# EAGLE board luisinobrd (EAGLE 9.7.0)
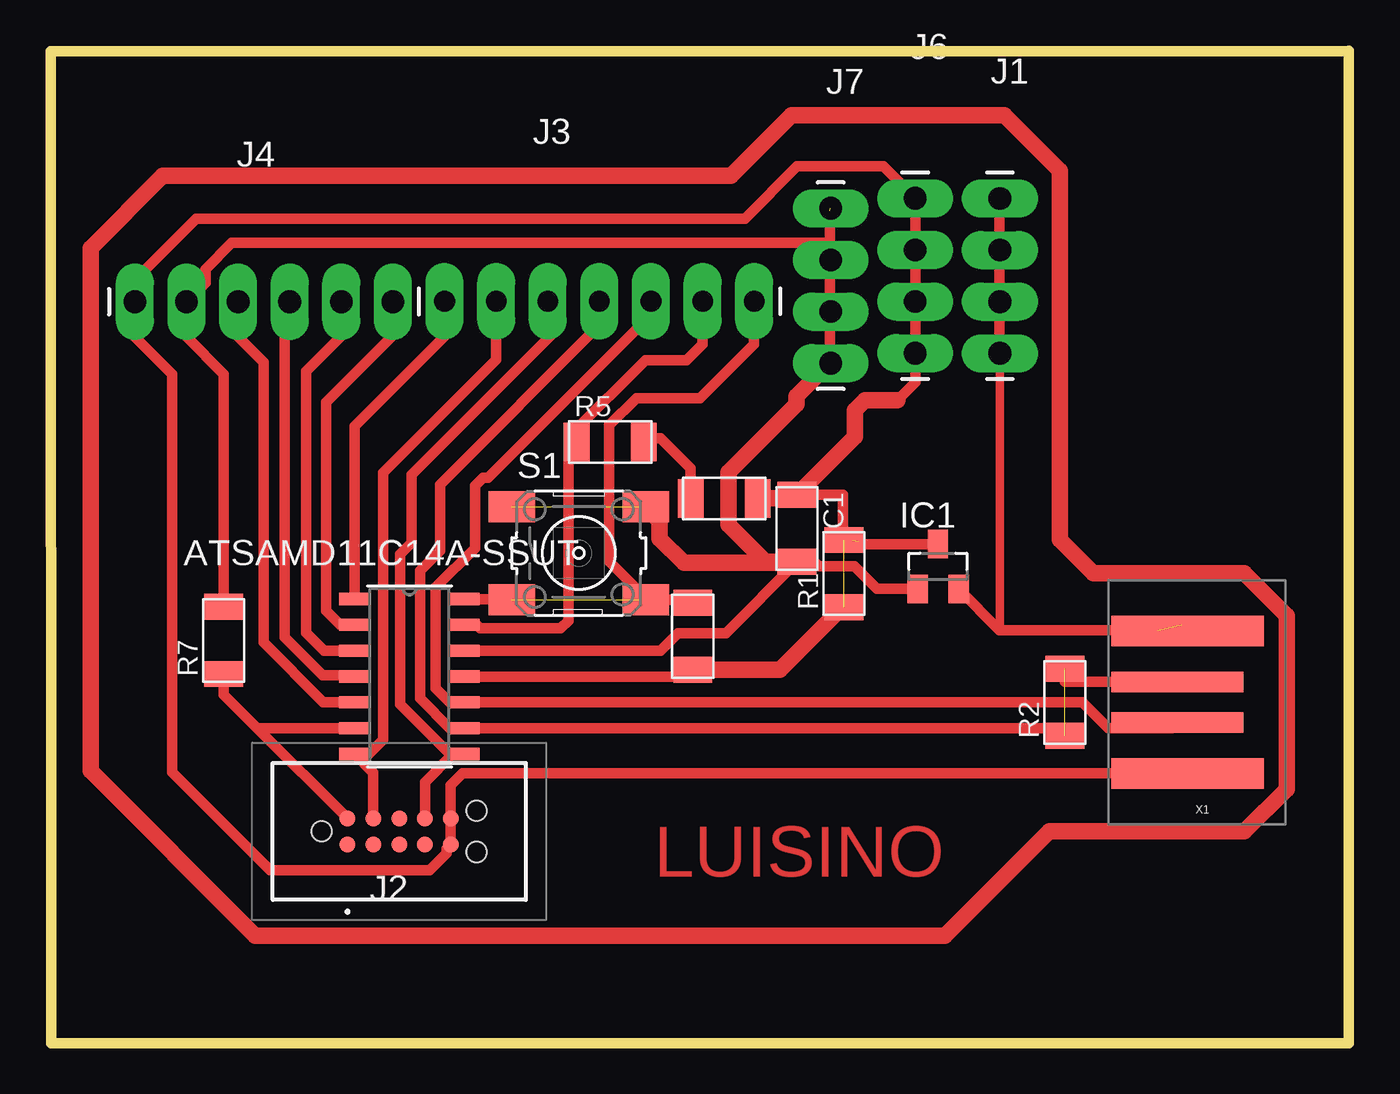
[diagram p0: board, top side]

Size 63.88 x 48.82 mm. Coordinates in mm from the lower left corner, seen from the top.
Outline: 63.88,48.82 63.88,0 0.02,0 0,48.79 63.88,48.79
Copper layers (1*16): Top / Bottom
Stack-up Default Layer Stack: Top User Defined 0.035mm / Dielectric-1 User Defined 1.5mm / Bottom User Defined 0.035mm
Design rules "default *": minimum track width 16mil, minimum drill 0.35mm, track to track 10mil, track to pad 16mil, pad to pad 16mil, via to via 16mil, smd to smd 6mil, copper to edge 16mil, drill to drill 16mil, minimum pad ring 10mil, minimum via ring 8mil, stop-mask expansion 4mil, vias tented up to drill 0mil, thermal gap 10mil

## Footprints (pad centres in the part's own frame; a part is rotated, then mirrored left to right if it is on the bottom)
C1206FAB = smd 1.27 x 1.905: 1 -1.651,0; 2 1.651,0
SOT23 = smd 1 x 1.4: 1 -1.001,-1.1; 2 1.014,-1.1; 3 0,1.1
1X04_LONGPADS = drill 1.118 pad 1.88 long: 1 0,0; 2 2.54,0; 3 5.08,0; 4 7.62,0
TC2050IDCNL = smd 0.787 x 0.787: 1 -2.54,-0.635; 2 -1.27,-0.635; 3 0,-0.635; 4 1.27,-0.635; 5 2.54,-0.635; 6 2.54,0.635; 7 1.27,0.635; 8 0,0.635; 9 -1.27,0.635; 10 -2.54,0.635 | hole 0.991: -3.81,0; 3.81,-1.015; 3.81,1.015
1X07_LONGPADS = drill 1.016 pad 1.88 long: 1 0,0; 2 2.54,0; 3 5.08,0; 4 7.62,0; 5 10.16,0; 6 12.7,0; 7 15.24,0
1X06_LONGPADS = drill 1.118 pad 1.88 long: 1 0,0; 2 2.54,0; 3 5.08,0; 4 7.62,0; 5 10.16,0; 6 12.7,0
R1206FAB = smd 1.27 x 1.905: 1 -1.651,0; 2 1.651,0
6MM_SWITCH = smd 2.286 x 1.524: 1 -3.302,2.286; 2 3.302,2.286; 3 -3.302,-2.286; 4 3.302,-2.286
SOIC14_SL_MCH = smd 1.5 x 0.6: 1 -2.7,3.81; 2 -2.7,2.54; 3 -2.7,1.27; 4 -2.7,0; 5 -2.7,-1.27; 6 -2.7,-2.54; 7 -2.7,-3.81; 8 2.7,-3.81; 9 2.7,-2.54; 10 2.7,-1.27; 11 2.7,0; 12 2.7,1.27; 13 2.7,2.54; 14 2.7,3.81
LED1206FAB = smd 1.27 x 1.905: 1 -1.651,0; 2 1.651,0
USB-A-PCB = smd 7.5 x 1.5: 5V -0.2,-3.5; GND -0.2,3.5 | smd 6.5 x 1: USB_M 0.3,-1; USB_P 0.3,1

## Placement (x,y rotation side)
C1  1uF  [C1206FAB]  36.73,25.32 270 top
IC1  [SOT23]  43.66,23.44 0 top
J1  [1X04_LONGPADS]  46.71,41.55 270 top
J2  TC2050-IDC-NL  [TC2050IDCNL]  17.14,10.41 0 top
J3  [1X07_LONGPADS]  19.38,36.5 0 top
J4  [1X06_LONGPADS]  4.14,36.47 0 top
J6  [1X04_LONGPADS]  42.55,41.56 270 top
J7  [1X04_LONGPADS]  38.38,41.07 270 top
R1  0  [R1206FAB]  39.04,23.1 90 top
R2  0  [R1206FAB]  49.91,16.76 90 top
R5  470  [R1206FAB]  27.53,29.57 0 top
R6  1k  [R1206FAB]  31.6,20.02 270 top
R7  10K  [R1206FAB]  8.51,19.81 90 top
S1  [6MM_SWITCH]  25.98,24.1 0 top
U1  ATSAMD11C14A-SSUT  [SOIC14_SL_MCH]  17.65,18.03 0 top
U$4  LEDFAB1206  [LED1206FAB]  33.15,26.8 0 top
X1  CONN_USBPCB  [USB-A-PCB]  55.75,16.76 180 top

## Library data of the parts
C1 IC1 R1 R2 R5-R7 S1 U$4 X1 = fab
J1 J6 J7 = SparkFun-Connectors; PROD_ID: CONN-09696
J2 = TC2050-IDC-NL; DESCRIPTION: 10-Pin No-Legs Plug-of-Nails Cable with Ribbon connector. CBL PLUG-OF-NAILS 10-PIN; HEIGHT: 29.66mm; MANUFACTURER_NAME: Tag-Connect; MANUFACTURER_PART_NUMBER: TC2050-IDC-NL
J3 J4 = SparkFun-Connectors
U1 = samd11c; BUILT_BY: EMA_Molly; COPYRIGHT: Copyright (C) 2018 Accelerated Designs. All rights reserved; MANUFACTURER_PART_NUMBER: ATSAMD11C14A-SSUT; SOURCELIBRARY: Microchip_2019-08-23_25; VENDOR: Microchip

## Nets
2: J3.6 R5.1 U1.13
4: J3.7 R6.1 S1.3 S1.4 U1.14
5: J3.1 U1.1
5V: IC1.2 J1.1 J1.2 J1.3 J1.4 X1.5V
8: J4.6 U1.2
9: J4.5 U1.3
24-: J3.4 R2.1 R2.2 U1.9 X1.USB_M
25+: J3.5 U1.10 X1.USB_P
CLK: J2.9 J3.2 U1.7
DIO: J2.7 J3.3 U1.8
GND: C1.1 IC1.3 J2.5 J2.6 J4.1 J6.1 J6.2 J6.3 J6.4 R1.1 R1.2 R6.2 U1.11 U$4.2 X1.GND
N$5: R5.2 U$4.1
RST: J2.10 R7.1 U1.6
SCL: J4.3 U1.5
SDA: J4.4 U1.4
VDD: C1.2 IC1.1 J4.2 J7.1 J7.2 J7.3 J7.4 R7.2 S1.1 S1.2 U1.12

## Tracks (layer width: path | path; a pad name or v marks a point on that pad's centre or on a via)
2
  Top 0.508: U1.13 20.96,20.57 21.14,20.4 25.09,20.4 25.48,20.78 25.48,29.49 25.81,29.49 R5.1 25.63,29.82 25.63,29.97 29.26,33.6 31.3,33.6 32.08,34.39 J3.6
4  (1 unrouted)
  Top 0.508: S1.4 31.45,21.82 R6.1 | S1.3 22.66,21.84 U1.14 | 28.99,21.82 S1.4 | S1.4 29.29,21.9 27.48,23.7 27.48,30.39 28.82,31.73 31.96,31.73 34.62,34.39 J3.7
5
  Top 0.508: J3.1 19.38,34.77 14.95,30.34 U1.1
5V  (1 unrouted)
  Top 0.406: X1.5V 55.64,20.57 | J1.4 46.71,20.33 46.7,20.32
  Top 0.508: 54.48,20.32 46.7,20.32 IC1.2 | 46.69,39.01 46.69,36.47 | J1.2 46.69,39.01 | J1.3 46.69,36.47 | 46.69,36.47 46.69,33.96 J1.4 47.22,33.43 | 46.69,39.01 46.69,41.53 J1.1
8
  Top 0.508: 15.01,20.63 U1.2 14.24,20.57 13.54,21.27 13.54,31.52 16.81,34.8 16.81,36.45 J4.6
9
  Top 0.508: U1.3 13.46,19.3 12.57,20.19 12.57,33.05 14.3,34.77 J4.5
24-  (1 unrouted)
  Top 0.406: U1.9 20.19,15.49 | 49.53,15.49 R2.1
  Top 0.508: U1.9 49.53,15.49 | R2.2 49.91,17.76 X1.USB_M | U1.9 20.29,15.43 | J3.4 27,35.33 19.15,27.48 19.15,24.21 18.18,23.24 18.18,16.95 19.66,15.47 20.33,15.47 U1.9
25+
  Top 0.406: X1.USB_P 55.18,15.49
  Top 0.508: J3.5 29.54,35.84 21.52,27.81 21.27,27.81 20.88,27.43 20.88,24.35 18.94,22.42 18.94,17.46 19.66,16.74 20.33,16.74 U1.10 50.78,16.76 52.05,15.49 55.18,15.49
CLK
  Top 0.508: J2.9 15.87,13.3 U1.7 | U1.7 15.02,14.15 | U1.7 14.97,14.2 15.65,14.2 16.36,14.92 16.36,28.06 21.92,33.61 J3.2
DIO
  Top 0.508: J2.7 18.41,12.84 19.76,14.18 20.31,14.18 U1.8 19.64,14.22 17.19,16.67 17.19,24.04 17.76,24.6 17.76,27.96 24.79,35 24.79,36.17 J3.3
GND  (2 unrouted)
  Top 0.406: 55.64,12.95 X1.GND
  Top 0.508: U1.11 31.27,18.03 R6.2 | X1.GND 21.38,13.26 | 21.38,13.26 | 21.38,13.26 20.26,13.26 19.69,12.69 J2.6 J2.5 19.47,9.56 19.47,9.34 18.63,8.51 10.79,8.51 5.97,13.34 5.97,32.92 4.14,34.75 J4.1 | 4.12,36.5 J4.1 | J4.1 4.14,37.54 7.16,40.56 34.16,40.56 36.73,43.13 40.98,43.13 J6.1 J6.2 J6.3 J6.4 42.55,32.5 41.66,31.62 | C1.1 38.99,26.98 38.99,24.8 R1.2 | 39.74,24.69 39.88,24.54 IC1.3
  Top 0.813: U$4.2 36.55,26.8 C1.1 39.59,29.83 39.59,31.14 40.06,31.62 41.66,31.62 | R6.2 35.89,18.36 38.97,21.45 R1.1 | 39.45,24.75 R1.2
N$1
  Top 0.813: 46.94,45.64 36.45,45.64 33.48,42.67 5.51,42.67 1.96,39.12 1.96,13.39 10.06,5.28 44.02,5.28 49.15,10.41 58.75,10.41 60.83,12.5 60.83,21.03 58.75,23.11 51.31,23.11 49.66,24.77 49.66,42.93 46.94,45.64
N$5
  Top 0.508: R5.2 29.39,29.77 30.02,29.77 31.5,28.29 U$4.1
RST
  Top 0.508: J2.10 10.16,15.49 | R7.1 8.51,17.15 10.16,15.49 | 10.16,15.49 U1.6
SCL
  Top 0.508: U1.5 13.42,16.76 10.47,19.71 10.47,33.5 9.22,34.75 J4.3
SDA
  Top 0.508: U1.4 14.9,18.09 13.38,18.09 11.51,19.96 11.51,36.23 J4.4
VDD  (2 unrouted)
  Top 0.508: 29.03,26.39 S1.2 29.79,25.88 | C1.2 36.47,23.67 | 38.35,38.41 38.35,35.94 | 38.35,40.95 38.35,39.37 | 38.35,39.37 38.35,38.41 | J7.4 38.35,33.48 38.35,35.94 | 38.35,38.41 38.38,38.43 J7.2 | 38.35,35.94 38.38,35.97 J7.3 | R7.2 8.51,32.92 6.68,34.75 J4.2 7.62,37.41 7.62,38.08 8.91,39.37 38.35,39.37 | C1.2 37.59,23.67 37.81,23.45 39.55,23.45 40.66,22.34 IC1.1 | U1.12 30.02,19.3 30.88,20.17 33.22,20.17 C1.2
  Top 0.813: 38.35,33.48 36.7,31.83 36.7,31.44 33.35,28.09 33.35,25.51 35.19,23.67 C1.2 37.16,23.67 37.21,23.62 31.17,23.62 29.97,24.82 29.97,25.71 S1.2

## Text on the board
Top: LUISINO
